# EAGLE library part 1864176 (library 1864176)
Phoenix Contact SDC Series 5mm Pitch, 16 Way Straight, PCB Terminal Block, SKEDD Source: Datasheet
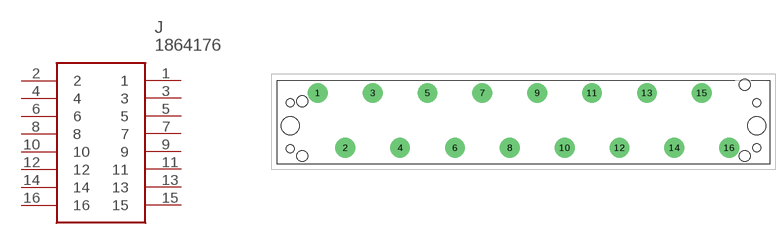
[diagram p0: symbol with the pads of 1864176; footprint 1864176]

Designator prefix J

## 1864176 (Arrow_Part_Number: 1864176; Arrow_Price-Stock: https://www.arrow.com/en/products/1864176/phoenix-contact; Description: Phoenix Contact SDC Series 5mm Pitch, 16 Way Straight, PCB Terminal Block, SKEDD; Height: 16mm; Manufacturer_Name: Phoenix Contact; Manufacturer_Part_Number: 1864176; Mouser_Part_Number: 651-1864176; Mouser_Price-Stock: https://www.mouser.com/Search/Refine.aspx?Keyword=651-1864176)  [1864176]
1  1
2  2
3  3
4  4
5  5
6  6
7  7
8  8
9  9
10  10
11  11
12  12
13  13
14  14
15  15
16  16

## Footprint 1864176 (pad centres in mm)
1864176
drill 2.4 pad 3.6: 1 -37.5,5.35; 2 -32.5,-4.65; 3 -27.5,5.35; 4 -22.5,-4.65; 5 -17.5,5.35; 6 -12.5,-4.65; 7 -7.5,5.35; 8 -2.5,-4.65; 9 2.5,5.35; 10 7.5,-4.65; 11 12.5,5.35; 12 17.5,-4.65; 13 22.5,5.35; 14 27.5,-4.65; 15 32.5,5.35; 16 37.5,-4.65
hole 3.3 at -42.5,-0.65
hole 3.3 at 42.5,-0.65
hole 2 at -40.3,3.85
hole 2 at -40.3,-6.15
hole 2 at 40.3,-6.15
hole 2 at 40.3,6.85
hole 1.5 at -42.5,3.55
hole 1.5 at -42.5,-4.85
hole 1.5 at 42.5,3.55
hole 1.5 at 42.5,-4.65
